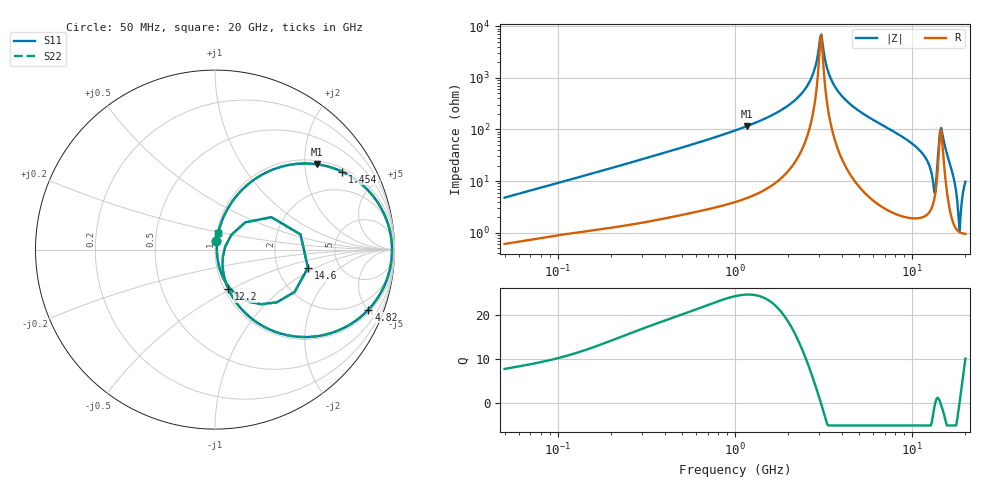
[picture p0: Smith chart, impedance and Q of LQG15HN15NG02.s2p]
!Murata Part Number: LQG15HN15NG02
!These Parameters are Measured in Series Mode Connection
!  o--[Z]--o
!Port1  Port2
!  o-------o
!Freq. Start=50[MHz] Stop=20[GHz], 401[Steps]
# Hz S RI R 50
!Freq.(Hz) S11(Real) S11(Imag) S21(Real) S21(Imag) S12(Real) S12(Imag) S22(Real) S22(Imag)
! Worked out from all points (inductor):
!   401 points, 50 MHz to 20 GHz, reference 50 ohm
!   read as one part in series: L = 14.9 nH near 51.52 MHz
!   highest Q = 24.7 at 1.162 GHz (marker M1), where L = 15.8 nH
!   self-resonance near 3.03 GHz
!   S11 on the Smith chart (normalised r, x): 50 MHz: 1.01, +0.10; 1.454 GHz: 1.13, +3.17; 4.82 GHz: 1.19, -5.04; 12.2 GHz: 1.05, -0.49; 14.6 GHz: 2.97, -0.84; 20 GHz: 1.02, +0.19
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5e7  0.00825 0.0468  0.9917 -0.0468  0.9917 -0.0468  0.00825 0.0468
1.364002e8  0.0248 0.1188  0.9752 -0.1188  0.9752 -0.1188  0.0248 0.1188
3.721004e8  0.1108 0.2878  0.8892 -0.2878  0.8892 -0.2878  0.1108 0.2878
1e9  0.4769 0.4793  0.5231 -0.4793  0.5231 -0.4793  0.4769 0.4793
1.161586e9  0.5673 0.4756  0.4327 -0.4756  0.4327 -0.4756  0.5673 0.4756
1.454215e9  0.7074 0.4346  0.2926 -0.4346  0.2926 -0.4346  0.7074 0.4346
2.179053e9  0.9178 0.2449  0.0822 -0.2449  0.0822 -0.2449  0.9178 0.2449
2.728004e9  0.9776 0.088  0.0224 -0.088  0.0224 -0.088  0.9776 0.088
3.075291e9  0.9862 -0.0038  0.0138 0.0038  0.0138 0.0038  0.9862 -0.0038
3.572216e9  0.9717 -0.1205  0.0283 0.1205  0.0283 0.1205  0.9717 -0.1205
4.81993e9  0.855 -0.3342  0.145 0.3342  0.145 0.3342  0.855 -0.3342
7.442007e9  0.508 -0.4872  0.492 0.4872  0.492 0.4872  0.508 -0.4872
1.019291e10  0.2125 -0.3907  0.7875 0.3907  0.7875 0.3907  0.2125 -0.3907
1.220001e10  0.0747 -0.2206  0.9253 0.2206  0.9253 0.2206  0.0747 -0.2206
1.334722e10  0.0443 -0.0376  0.9557 0.0376  0.9557 0.0376  0.0443 -0.0376
1.396067e10  0.1687 0.1519  0.8313 -0.1519  0.8313 -0.1519  0.1687 0.1519
1.460232e10  0.5177 -0.1014  0.4823 0.1014  0.4823 0.1014  0.5177 -0.1014
1.527346e10  0.2584 -0.3045  0.7416 0.3045  0.7416 0.3045  0.2584 -0.3045
1.670968e10  0.0441 -0.1545  0.9559 0.1545  0.9559 0.1545  0.0441 -0.1545
1.828096e10  0.0108 -0.0172  0.9892 0.0172  0.9892 0.0172  0.0108 -0.0172
1.88369e10  0.0104 0.022  0.9896 -0.022  0.9896 -0.022  0.0104 0.022
2e10  0.0185 0.0944  0.9815 -0.0944  0.9815 -0.0944  0.0185 0.0944
